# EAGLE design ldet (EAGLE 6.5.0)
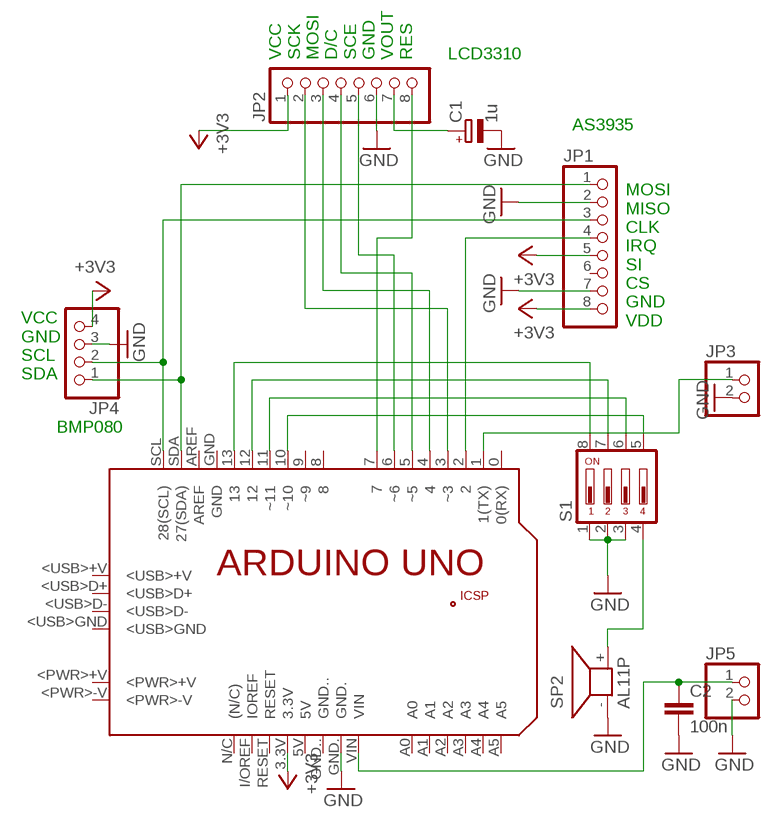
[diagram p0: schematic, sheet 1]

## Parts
C1  1u  CPOL-EUTT2D4L  [TT2D4L]
C2  100n  C-EU050-024X044  [C050-024X044]
JP1  PINHD-1X8  [1X08]
JP2  PINHD-1X8  [1X08]
JP3  PINHD-1X2/90  [1X02/90]
JP4  PINHD-1X4  [1X04]
JP5  PINHD-1X2/90  [1X02/90]
PCB1  ARDUINO_UNO  [ARDUINO_UNO]
S1  DIP04YL  [DIP04YL]
SP2  AL11P  [AL11P]

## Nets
+3V3: JP1.5 JP1.8 JP2.1 JP4.4 PCB1.3.3V
GND: C1.- C2.2 JP1.2 JP1.7 JP2.6 JP3.2 JP4.3 JP5.2 PCB1.GND. S1.1 S1.2 S1.3 SP2.-
N$1: JP1.4 PCB1.2
N$2: JP1.3 JP4.2 PCB1.SCL(28(SCL))
N$3: JP1.1 JP4.1 PCB1.SDA(27(SDA))
N$4: C1.+ JP2.7
N$5: JP2.8 PCB1.7
N$6: JP2.5 PCB1.6(~6)
N$7: JP2.4 PCB1.5(~5)
N$8: JP2.3 PCB1.4
N$9: JP2.2 PCB1.3(~3)
N$10: S1.4 SP2.+
N$11: PCB1.12 S1.7
N$12: PCB1.11(~11) S1.6
N$13: PCB1.13 S1.8
N$14: PCB1.10(~10) S1.5
N$15: JP3.1 PCB1.1(1(TX))
N$20: C2.1 JP5.1 PCB1.VIN
Unconnected: JP1.6 PCB1.0(0(RX)) PCB1.5V PCB1.8 PCB1.9(~9) PCB1.+5V PCB1.<PWR>+V PCB1.<PWR>-V PCB1.<USB>+V PCB1.<USB>D+ PCB1.<USB>D- PCB1.<USB>GND PCB1.A0 PCB1.A1 PCB1.A2 PCB1.A3 PCB1.A4 PCB1.A5 PCB1.AREF PCB1.GND PCB1.GND.. PCB1.GND_ PCB1.I/OREF(IOREF) PCB1.MISO PCB1.MOSI PCB1.N/C((N/C)) PCB1.RESET PCB1.RESET. PCB1.SCK

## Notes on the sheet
- VCC
  SCK
  MOSI
  D/C
  SCE
  GND
  VOUT
  RES
- LCD3310
- AS3935
- MOSI
  MISO
  CLK
  IRQ
  SI
  CS
  GND
  VDD
- VCC
  GND
  SCL
  SDA
- BMP080

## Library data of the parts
C1 = rcl:CPOL-EU: POLARIZED CAPACITOR, European symbol
C2 = rcl:C-EU: CAPACITOR, European symbol
JP1 JP2 = pinhead:PINHD-1X8: PIN HEADER
JP3 JP5 = pinhead:PINHD-1X2: PIN HEADER
JP4 = pinhead:PINHD-1X4: PIN HEADER
PCB1 = Arduino_revB:ARDUINO_UNO: Device for representing an Arduino Uno board with a footprint in an EAGLE design. Created by Dave Young for Element14. More EAGLE documentation at: http://www.element14.com/community/community/knode/cadsoft_eagle
S1 = switch-dil:DIP04YL: DIL/CODE SWITCH; OC_FARNELL: unknown; OC_NEWARK: unknown
SP2 = buzzer:AL11P: SPEAKER; OC_FARNELL: unknown; OC_NEWARK: unknown

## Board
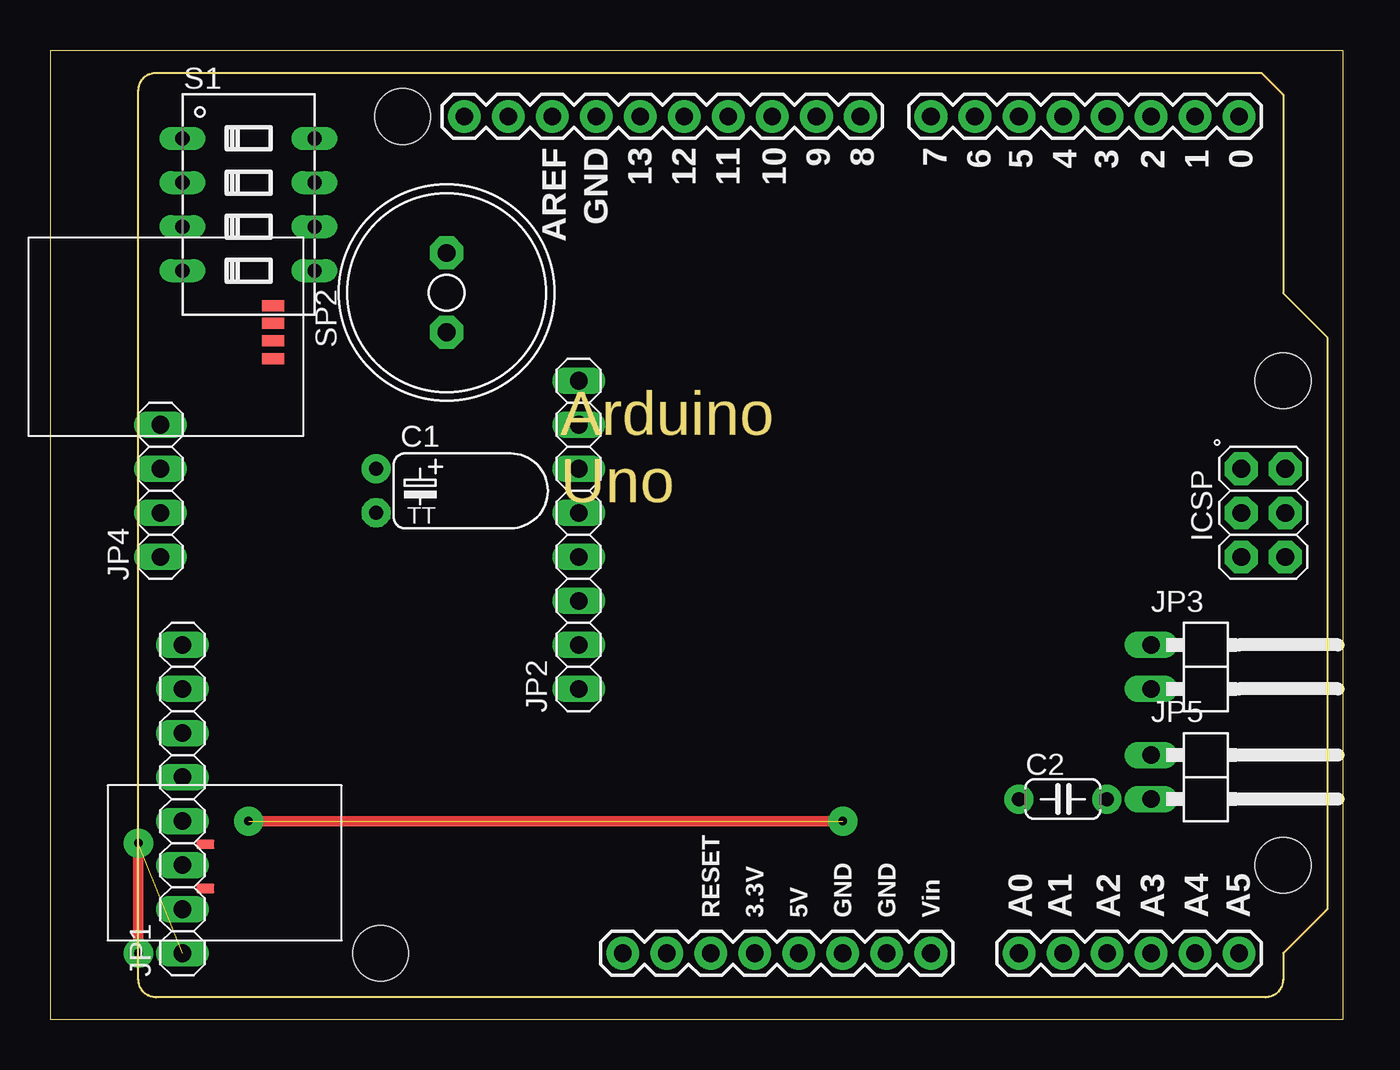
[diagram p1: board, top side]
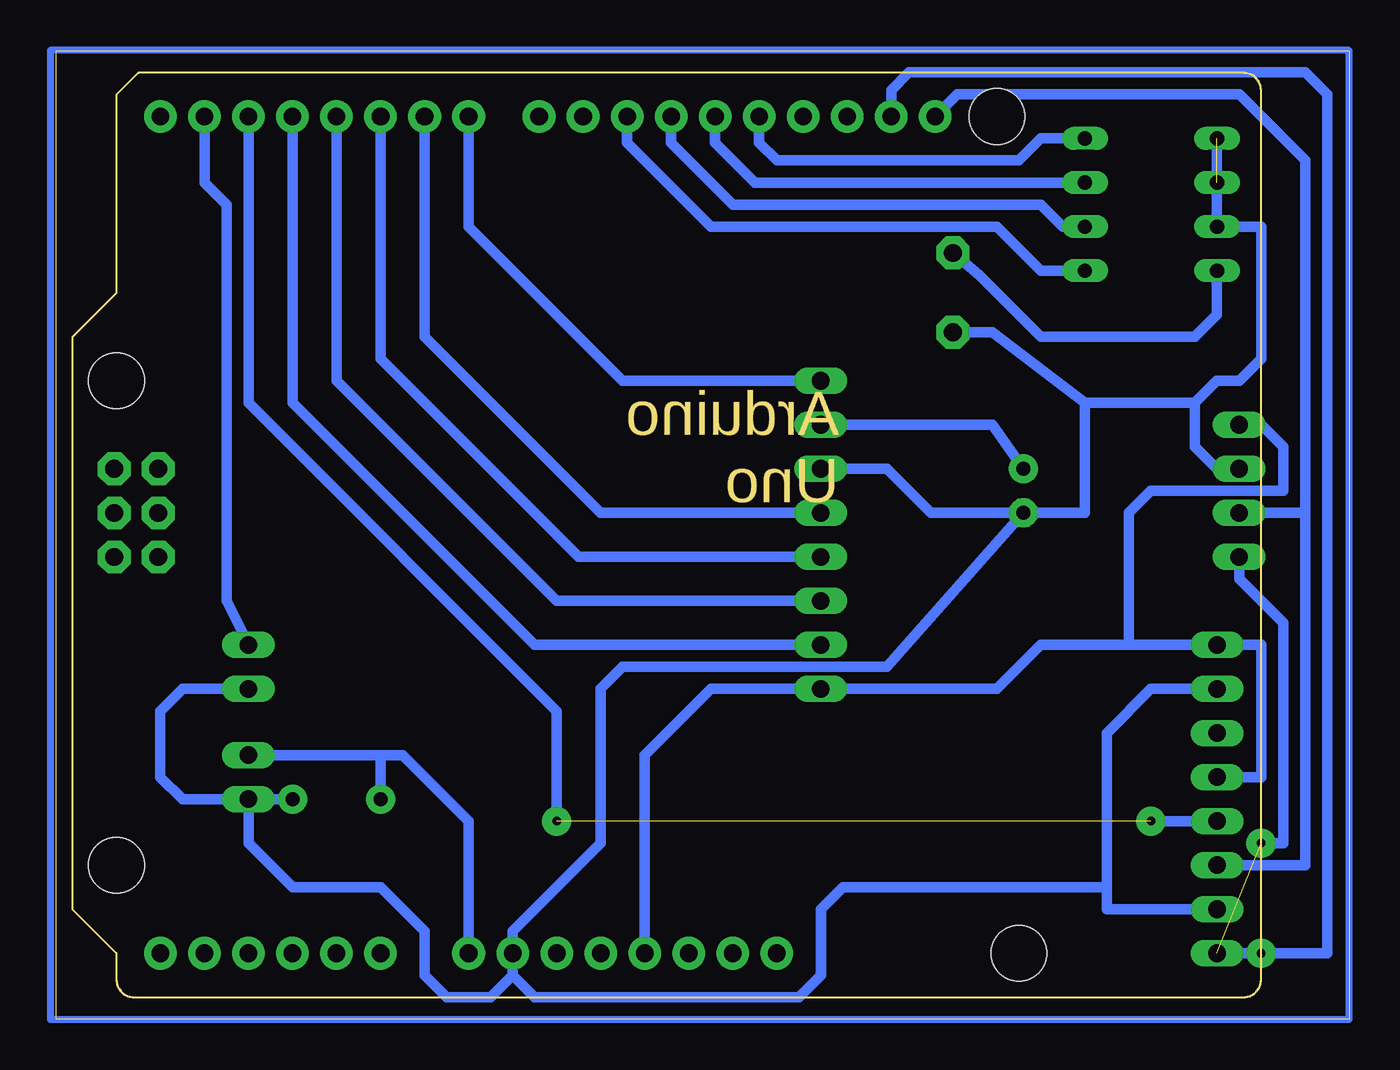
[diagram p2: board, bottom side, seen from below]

Size 74.6 x 55.87 mm. Coordinates in mm from the lower left corner, seen from the top.
Outline: 0,0 74.6,0 74.6,55.87 0,55.87 0,0
Copper layers (1*16): Top 0.035mm / dielectric 1.5mm / Bottom 0.035mm
Design rules "default": minimum track width 10mil, minimum drill 24mil, track to track 8mil, track to pad 8mil, pad to pad 8mil, via to via 8mil, smd to smd 8mil, copper to edge 40mil, drill to drill 8mil, minimum pad ring 10mil, minimum via ring 8mil, stop-mask expansion 4mil, vias tented up to drill 0mil, thermal gap 10mil

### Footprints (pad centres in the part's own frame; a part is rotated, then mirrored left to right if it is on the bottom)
TT2D4L = drill 0.813 pad 1.6: + -1.27,0 | drill 0.813 pad 1.6 octagon: - 1.27,0
C050-024X044 = drill 0.813 octagon: 1 -2.54,0; 2 2.54,0
1X08 = drill 1.016 long: 1 -8.89,0; 2 -6.35,0; 3 -3.81,0; 4 -1.27,0; 5 1.27,0; 6 3.81,0; 7 6.35,0; 8 8.89,0
1X02/90 = drill 1.016 long: 1 -1.27,-3.81; 2 1.27,-3.81
1X04 = drill 1.016 long: 1 -3.81,0; 2 -1.27,0; 3 1.27,0; 4 3.81,0
ARDUINO_UNO = drill 1.016 pad 1.88: 0 63.5,50.8; 1 60.96,50.8; 2 58.42,50.8; 3 55.88,50.8; 3.3V 35.56,2.54; 4 53.34,50.8; 5 50.8,50.8; 5V 38.1,2.54; 6 48.26,50.8; 7 45.72,50.8; 8 41.656,50.8; 9 39.116,50.8; 10 36.576,50.8; 11 34.036,50.8; 12 31.496,50.8; 13 28.956,50.8; A0 50.8,2.54; A1 53.34,2.54; A2 55.88,2.54; A3 58.42,2.54; A4 60.96,2.54; A5 63.5,2.54; AREF 23.876,50.8; GND 26.416,50.8; GND. 43.18,2.54; GND.. 40.64,2.54; I/OREF 30.48,2.54; N/C 27.94,2.54; RESET 33.02,2.54; SCL 18.796,50.8; SDA 21.336,50.8; VIN 45.72,2.54 | drill 1.016 pad 1.88 octagon: +5V 66.167,30.48; GND_ 66.167,25.4; MISO 63.627,30.48; MOSI 66.167,27.94; RESET. 63.627,25.4; SCK 63.627,27.94 | smd 1.016 x 0.508: <PWR>+V 3.861,8.814; <PWR>-V 3.861,6.274 | smd 1.27 x 0.635: <USB>+V 7.772,39.878; <USB>D+ 7.772,38.887; <USB>D- 7.772,37.871; <USB>GND 7.772,36.83 | hole 3.2: 66.04,7.62; 66.04,35.56; 15.24,50.8; 13.97,2.54
DIP04YL = drill 0.813 long: 1 -3.81,-3.81; 2 -1.27,-3.81; 3 1.27,-3.81; 4 3.81,-3.81; 5 3.81,3.81; 6 1.27,3.81; 7 -1.27,3.81; 8 -3.81,3.81
AL11P = drill 1.016 pad 1.905 octagon: + 2.286,0; - -2.286,0

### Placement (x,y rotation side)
C1  18.8,30.48 270 top
C2  58.42,12.7 0 top
JP1  7.62,12.7 90 top
JP2  30.48,27.94 90 top
JP3  67.31,20.32 270 top
JP4  6.35,30.48 90 top
JP5  67.31,13.97 270 top
PCB1  5.08,1.27 0 top
S1  11.43,46.99 270 top
SP2  22.86,41.91 90 top

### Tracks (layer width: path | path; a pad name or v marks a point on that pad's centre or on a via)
+3V3
  Bottom 0.61: PCB1.3.3V 40.64,15.24 36.83,19.05 JP2.1 20.32,19.05 17.78,21.59 12.7,21.59 | JP1.5 5.08,13.97 5.08,21.59 JP1.8 12.7,21.59 | JP4.4 5.08,34.29 3.81,33.02 3.81,30.48 11.43,30.48 12.7,29.21 12.7,21.59
GND  (1 unrouted)
  Bottom 0.61: S1.1 S1.3 5.08,45.72 5.08,38.1 6.35,36.83 7.62,36.83 8.89,35.56 | C1.- 26.67,20.32 41.91,20.32 43.18,19.05 43.18,10.16 48.26,5.08 PCB1.GND. 48.26,2.54 | JP1.7 11.43,19.05 13.97,16.51 13.97,7.62 | JP1.2 13.97,6.35 13.97,7.62 | 48.26,2.54 46.99,1.27 31.75,1.27 30.48,2.54 30.48,6.35 29.21,7.62 13.97,7.62 | C1.- 24.13,29.21 26.67,31.75 JP2.6 | SP2.- 20.57,39.62 15.24,35.56 | 15.24,35.56 15.24,29.21 C1.- | 8.89,35.56 15.24,35.56 | 8.89,35.56 8.89,33.02 7.62,31.75 JP4.3 | 48.26,2.54 49.53,1.27 52.07,1.27 53.34,2.54 53.34,5.08 55.88,7.62 60.96,7.62 63.5,10.16 JP5.2 | JP3.2 67.31,19.05 68.58,17.78 68.58,13.97 67.31,12.7 JP5.2 | JP5.2 C2.2
N$1  (1 unrouted)
  Bottom 0.61: JP1.4 11.43,11.43 | PCB1.2 63.5,35.56 45.72,17.78 45.72,11.43
N$2
  Bottom 0.61: JP1.3 2.54,8.89 2.54,29.21 | 2.54,29.21 2.54,49.53 6.35,53.34 22.61,53.34 PCB1.SCL | JP4.2 2.54,29.21
N$3  (1 unrouted)
  Bottom 0.61: PCB1.SDA 26.42,53.59 25.4,54.61 2.54,54.61 1.27,53.34 1.27,3.81 JP1.1 | JP4.1 6.35,25.4 3.81,22.86 3.81,10.16 5.08,10.16
N$4
  Bottom 0.61: C1.+ 20.57,34.29 JP2.7
N$5
  Bottom 0.61: JP2.8 41.91,36.83 50.8,45.72 PCB1.7
N$6
  Bottom 0.61: JP2.5 43.18,29.21 53.34,39.37 PCB1.6
N$7
  Bottom 0.61: JP2.4 44.45,26.67 55.88,38.1 PCB1.5
N$8
  Bottom 0.61: JP2.3 45.72,24.13 58.42,36.83 PCB1.4
N$9
  Bottom 0.61: JP2.2 46.99,21.59 60.96,35.56 PCB1.3
N$10
  Bottom 0.61: S1.4 7.62,40.64 8.89,39.37 17.78,39.37 21.34,42.93 SP2.+
N$11
  Bottom 0.61: PCB1.12 36.58,50.55 34.29,48.26 S1.7
N$12
  Bottom 0.61: PCB1.11 39.12,50.55 35.56,46.99 17.78,46.99 16.51,45.72 S1.6
N$13
  Bottom 0.61: PCB1.13 34.04,50.55 33.02,49.53 19.05,49.53 17.78,50.8 S1.8
N$14
  Bottom 0.61: PCB1.10 41.66,50.55 36.83,45.72 20.32,45.72 17.78,43.18 S1.5
N$15
  Bottom 0.61: PCB1.1 66.04,48.26 64.77,46.99 64.77,24.13 JP3.1
N$16  (via drill 0.5 pad 1.68)
  Top 0.61: v5.08,10.16 v5.08,3.81
N$17  (via drill 0.5 pad 1.68)
  Top 0.61: v11.43,11.43 v45.72,11.43
N$18  (via drill 0.5 pad 1.68)
  other vias: 18.8,31.75
N$19  (via drill 0.5 pad 1.68)
  other vias: 18.8,29.21
N$20
  Bottom 0.61: PCB1.VIN 50.8,11.43 54.61,15.24 55.88,15.24 | 55.88,15.24 JP5.1 | C2.1 55.88,15.24
N$21  (via drill 0.5 pad 1.68)
  other vias: 55.88,12.7
N$22  (via drill 0.5 pad 1.68)
  other vias: 60.96,12.7
N$23  (via drill 0.9 pad 2.54)
  other vias: 71.12,36.83
N$24  (via drill 0.9 pad 2.54)
  other vias: 71.12,8.89
N$25  (via drill 0.9 pad 2.54)
  other vias: 19.05,3.81
N$26
  Bottom 0.406: 0,55.88 74.93,55.88 74.93,0 0,0 0,55.88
